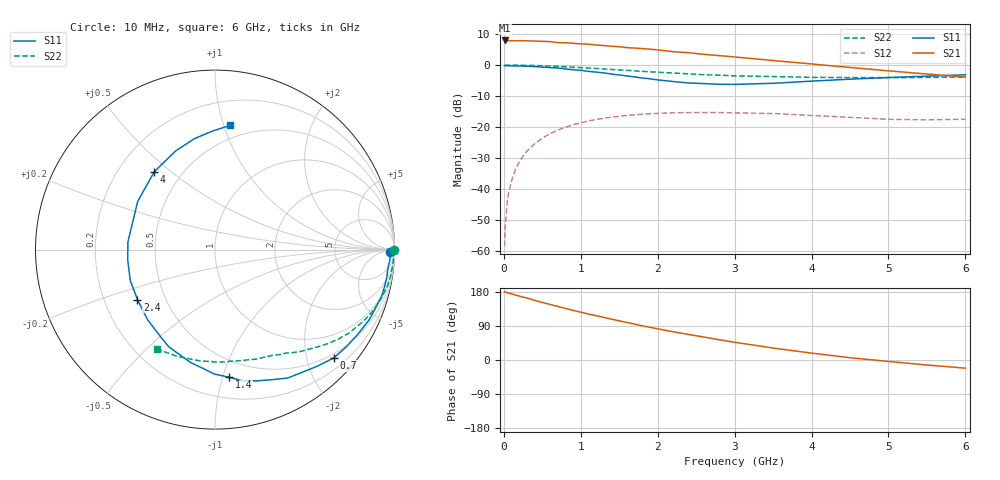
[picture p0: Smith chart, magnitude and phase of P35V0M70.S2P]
! SIEMENS Small Signal Semiconductors
! BFP181
! Si NPN RF Bipolar Junction Transistor in SOT143
! VCE = 5 V  IC = 0.7 mA
! Common Emitter S-Parameters:  March  1996
# GHz  S  MA  R  50
!  f  S11  S21  S12  S22
! GHz  MAG  ANG  MAG  ANG  MAG  ANG  MAG  ANG
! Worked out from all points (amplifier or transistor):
!   36 points, 10 MHz to 6 GHz, reference 50 ohm
!   highest |S21| = 7.9 dB at 10 MHz (marker M1)
!   |S21| within 3 dB of that: start of sweep to 1.977 GHz
!   unconditionally stable (mu >= 1): 3.578 GHz to end of sweep
!   at 250 MHz: K = 0.08, MSG = 18.6 dB, |S12| = -29.4 dB
!   at 1.4 GHz: K = 0.44, MSG = 11.4 dB, |S12| = -16.8 dB
!   at 6 GHz: K = 1.37, MAG = 3.2 dB, |S12| = -17.5 dB
!   S11 on the Smith chart (normalised r, x): 10 MHz: 55, -32; 700 MHz: 0.41, -2.53; 1.4 GHz: 0.36, -1.05; 2.4 GHz: 0.35, -0.26; 4 GHz: 0.35, +0.44; 6 GHz: 0.39, +1.05
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0.01  0.9734 -0.9  2.491 179.6  0.0012 86.3  0.9978 -0.2
0.02  0.9764 -1.2  2.476 179.5  0.0026 89.9  0.9967 -0.7
0.05  0.9769 -2.9  2.479 177.1  0.0073 92.2  0.9963 -1.5
0.1  0.9691 -6.3  2.472 174.5  0.0136 85.7  0.995 -3.0
0.15  0.9698 -9.3  2.458 171.5  0.0206 83.1  0.9947 -4.4
0.25  0.9646 -15.3  2.471 165.9  0.034 79.7  0.9902 -7.3
0.4  0.9441 -24.4  2.433 157.3  0.0537 73.3  0.9828 -11.6
0.6  0.9101 -36.6  2.389 146.6  0.0781 64.7  0.9619 -17.2
0.7  0.8956 -42.3  2.302 141.3  0.0891 61.1  0.9496 -19.9
0.8  0.866 -48.4  2.289 136.1  0.0991 57.0  0.9373 -22.4
1.1  0.7914 -66.3  2.169 121.2  0.1254 46.2  0.8931 -29.5
1.4  0.715 -83.8  2.009 107.8  0.1442 36.5  0.8488 -36.0
1.5  0.6936 -90.3  1.977 103.3  0.149 33.7  0.8331 -37.8
1.9  0.5998 -115.3  1.803 86.4  0.1635 23.4  0.7773 -44.8
2.2  0.5422 -133.8  1.645 74.5  0.1696 16.7  0.7435 -49.6
2.4  0.5141 -147.2  1.579 67.4  0.171 12.5  0.721 -52.7
3  0.4873 175.1  1.35 46.8  0.1695 2.2  0.6699 -61.6
3.5  0.5076 148.0  1.183 31.6  0.1653 -3.9  0.652 -69.3
4  0.5503 127.9  1.041 18.1  0.1539 -8.1  0.6328 -78.3
4.5  0.5911 112.0  0.913 6.1  0.1435 -10.9  0.6281 -88.4
5.5  0.6613 91.0  0.716 -13.2  0.1306 -7.0  0.631 -109.4
6  0.6969 83.1  0.64 -21.5  0.1337 -4.3  0.642 -120.3
